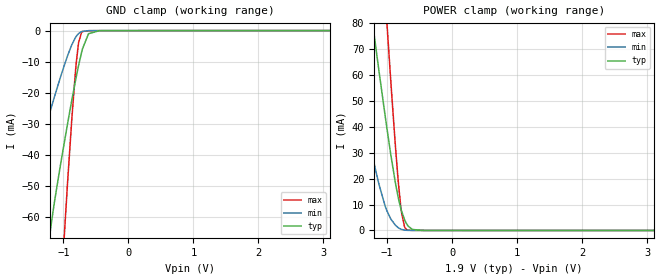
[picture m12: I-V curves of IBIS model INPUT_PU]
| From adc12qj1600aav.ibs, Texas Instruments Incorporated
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[Model]   INPUT_PU
Model_type   Input
Vinl = 0.45
Vinh = 0.7
|   typ   min   max
C_comp   0.62p   0.51p   0.71p
[Voltage Range]   1.9   1.8   2
[Temperature Range]   25   125   -40
[Power Clamp Reference]   1.9   1.8   2
[GND Clamp Reference]   0   0   0
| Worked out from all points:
|   GND clamp passes 1 mA (typ) near -0.61 V on its own axis
|   POWER clamp passes 1 mA (typ) near -0.64 V on its own axis
[GND Clamp]
|   Voltage   I(typ)   I(min)   I(max)
-1.8V     -213.8mA   -95.12mA   -502.1mA
-1.616V   -163.6mA   -66.05mA   -393.9mA
-1.4V     -107.1mA   -41mA      -268.6mA
-1.195V   -63.83mA   -25.54mA   -155mA
-1.033V   -42.02mA   -14.31mA   -82.71mA
-936mV    -30.21mA   -8.193mA   -49.51mA
-801mV    -14.93mA   -1.849mA   -10.46mA
-763.2mV  -11.08mA   -922.9uA   -3.76mA
-720mV    -7.133mA   -359.7uA   -639.3uA
-612mV    -1.012mA   -36.56uA   -30.82uA
-444.6mV  -25.34uA   -14.19uA   -25.73uA
3.6V      0A         0A         0A
[POWER Clamp]
|   Voltage   I(typ)   I(min)   I(max)
-1.8V     194.1mA    101.9mA    402.9mA
-1.4V     114.6mA    50.04mA    238.7mA
-1.287V   92.48mA    36.1mA     192.7mA
-1.184V   72.83mA    24.23mA    151.4mA
-1.001V   39.19mA    7.519mA    79.49mA
-871.2mV  18.36mA    2.048mA    32.55mA
-822.6mV  12.07mA    988.1uA    17.51mA
-779.4mV  7.674mA    431.6uA    7.221mA
-730.8mV  4.171mA    147.4uA    1.385mA
-676.8mV  1.74mA     46.74uA    132.1uA
-444.6mV  17.53uA    11.22uA    20.89uA
3.6V      0A         0A         0A
